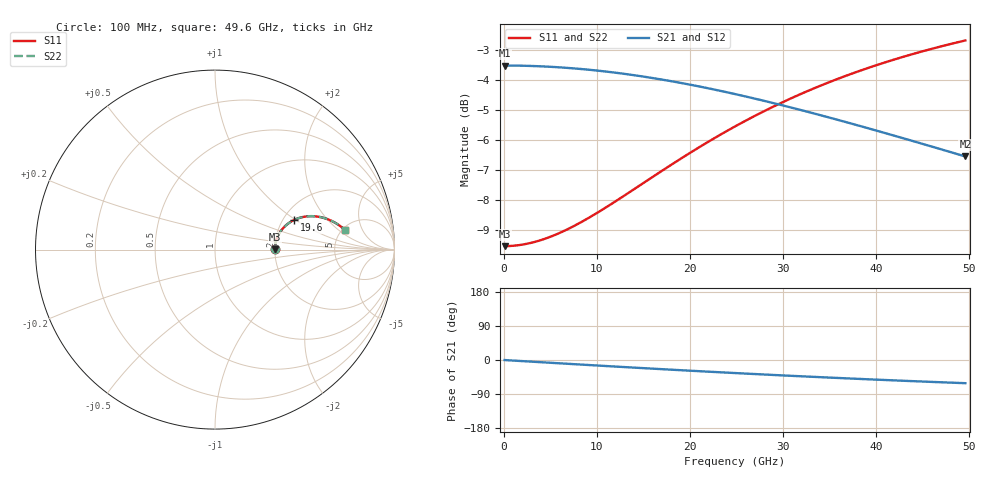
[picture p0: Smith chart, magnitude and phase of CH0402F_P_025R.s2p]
# GHz S RI R 25
! S-Parameters data
! Freq  reS11  imS11  reS21  imS21  reS12  imS12  reS22  imS22
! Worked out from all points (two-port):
!   100 points, 100 MHz to 49.6 GHz, reference 25 ohm
!   highest |S21| = -3.52 dB at 100 MHz (marker M1); lowest = -6.6 dB at 49.6 GHz (marker M2)
!   |S21| within 3 dB of the highest: start of sweep to 49.26 GHz
!   lowest |S11| = -9.5 dB at 100 MHz (marker M3), VSWR 2.00, Z = 50 + j0.121 ohm
!   |S11| at or under -10 dB: nowhere
!   |S22| runs from -9.5 to -2.7 dB; largest |S21 - S12| = 0
!   S11 on the Smith chart (normalised r, x): 100 MHz: 2.00, +0.00; 19.6 GHz: 2.29, +0.98; 49.6 GHz: 5.32, +2.49
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0.1  0.3333 0.00107  0.6667 -0.0017  0.6667 -0.0017  0.3333 0.00107
2.1  0.3348 0.0224  0.6651 -0.0356  0.6651 -0.0356  0.3348 0.0224
4.1  0.3388 0.0435  0.6609 -0.0692  0.6609 -0.0692  0.3388 0.0435
6.1  0.3453 0.0639  0.6539 -0.1022  0.6539 -0.1022  0.3453 0.0639
8.6  0.3569 0.088  0.6417 -0.142  0.6417 -0.142  0.3569 0.088
10.6  0.3686 0.1059  0.6292 -0.1724  0.6292 -0.1724  0.3686 0.1059
12.6  0.3822 0.1223  0.6146 -0.2014  0.6146 -0.2014  0.3822 0.1223
14.6  0.3977 0.1371  0.5981 -0.2286  0.5981 -0.2286  0.3977 0.1371
16.6  0.4146 0.15  0.58 -0.2541  0.58 -0.2541  0.4146 0.15
19.6  0.4423 0.1658  0.5502 -0.2885  0.5502 -0.2885  0.4423 0.1658
22.1  0.4669 0.1756  0.5235 -0.3137  0.5235 -0.3137  0.4669 0.1756
25.1  0.4976 0.1831  0.49 -0.3398  0.49 -0.3398  0.4976 0.1831
27.1  0.5185 0.1857  0.4671 -0.3547  0.4671 -0.3547  0.5185 0.1857
29.1  0.5394 0.1863  0.444 -0.3677  0.444 -0.3677  0.5394 0.1863
31.1  0.5601 0.1852  0.4209 -0.3788  0.4209 -0.3788  0.5601 0.1852
33.1  0.5806 0.1823  0.398 -0.3881  0.398 -0.3881  0.5806 0.1823
35.1  0.6007 0.1779  0.3752 -0.3958  0.3752 -0.3958  0.6007 0.1779
37.1  0.6203 0.1719  0.3529 -0.4019  0.3529 -0.4019  0.6203 0.1719
39.1  0.6392 0.1646  0.3311 -0.4066  0.3311 -0.4066  0.6392 0.1646
41.6  0.6619 0.1536  0.3045 -0.4106  0.3045 -0.4106  0.6619 0.1536
45.6  0.6956 0.1325  0.2641 -0.4133  0.2641 -0.4133  0.6956 0.1325
49.6  0.726 0.1078  0.2266 -0.4121  0.2266 -0.4121  0.726 0.1078
